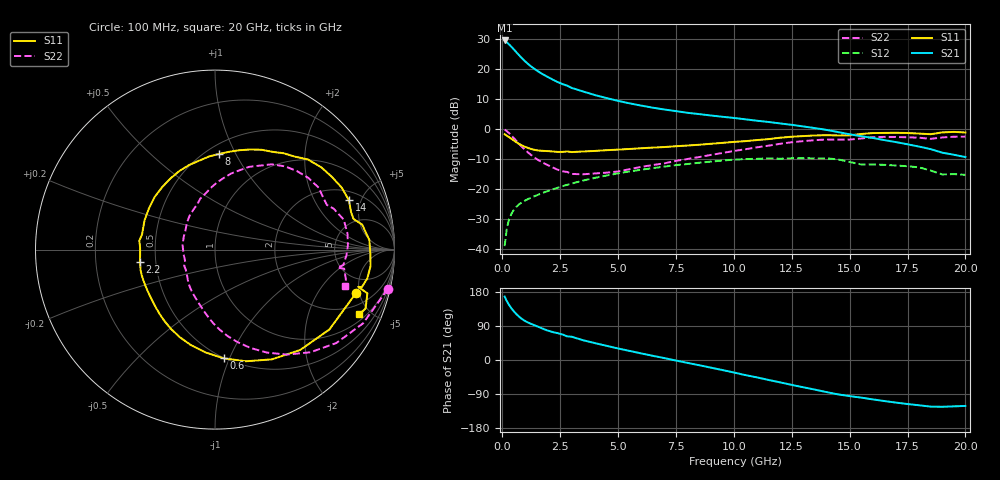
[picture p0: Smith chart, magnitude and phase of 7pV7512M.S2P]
! Infineon Technologies  Discrete & RF Semiconductors
! bfp620
! VCE = 0.75 V,  IC =  12 mA
! Common Emitter S-Parameters:  Sep 2002
# GHz  S  MA  R  50
!  f  S11  S21  S12  S22
! GHz  MAG  ANG  MAG  ANG  MAG  ANG  MAG  ANG
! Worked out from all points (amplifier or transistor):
!   59 points, 100 MHz to 20 GHz, reference 50 ohm
!   highest |S21| = 29.6 dB at 100 MHz (marker M1)
!   |S21| within 3 dB of that: start of sweep to 500.8 MHz
!   unconditionally stable (mu >= 1): 3.911 GHz to 10.42 GHz; 16.99 GHz to end of sweep
!   at 1 GHz: K = 0.55, MSG = 23.1 dB, |S12| = -23.7 dB
!   at 5.5 GHz: K = 1.05, MAG = 10.0 dB, |S12| = -14.1 dB
!   at 20 GHz: K = 1.49, MAG = -1.2 dB, |S12| = -15.2 dB
!   S11 on the Smith chart (normalised r, x): 100 MHz: 3.11, -4.64; 600 MHz: 0.50, -0.95; 2.2 GHz: 0.41, -0.07; 8 GHz: 0.58, +0.86; 14 GHz: 2.63, +3.93; 20 GHz: 1.33, -4.29
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0.1  0.8223 -17.1  30.16 167.3  0.0112 79.9  0.987 -12.9
0.2  0.7774 -34.9  27.99 154.8  0.0228 72.4  0.9215 -26.5
0.3  0.7335 -49.7  25.79 144.6  0.0319 66.6  0.8531 -37.6
0.4  0.6884 -62.7  23.55 135.9  0.0392 61.6  0.781 -47.1
0.5  0.6454 -74.6  21.37 128.3  0.0453 57.5  0.7097 -55.5
0.6  0.6075 -85.5  19.35 121.6  0.0504 54.2  0.643 -63.2
0.7  0.5754 -95.3  17.53 115.7  0.0547 51.5  0.5831 -70.1
0.8  0.5485 -104.2  15.94 110.5  0.0586 49.5  0.5307 -76.3
0.9  0.5256 -112.0  14.57 106.1  0.062 47.9  0.4854 -81.9
1.1  0.4884 -125.0  12.36 99.2  0.068 45.9  0.4124 -91.1
1.6  0.4395 -149.3  8.936 86.5  0.0822 43.3  0.2983 -109.9
2.2  0.424 -170.7  6.642 73.4  0.0999 40.5  0.2278 -131.7
2.8  0.4248 173.3  5.316 62.4  0.1181 37.2  0.1935 -152.5
3.5  0.425 157.6  4.242 51.9  0.1395 32.3  0.177 -172.7
5  0.4562 130.0  2.967 30.4  0.1834 20.1  0.1971 146.2
7  0.5036 100.0  2.128 5.0  0.2378 2.0  0.2693 111.9
8  0.5335 87.5  1.876 -7.6  0.2626 -8.1  0.3186 99.2
10.5  0.6317 59.6  1.46 -39.9  0.3174 -36.1  0.4627 72.8
13.5  0.7858 26.1  1.043 -78.2  0.3264 -70.2  0.6559 37.5
14  0.7951 20.2  0.974 -84.6  0.3264 -76.8  0.673 30.8
17  0.8712 -6.3  0.609 -112.4  0.2481 -100.9  0.7411 1.9
20  0.8815 -24.1  0.343 -121.2  0.1731 -112.7  0.7501 -15.7
